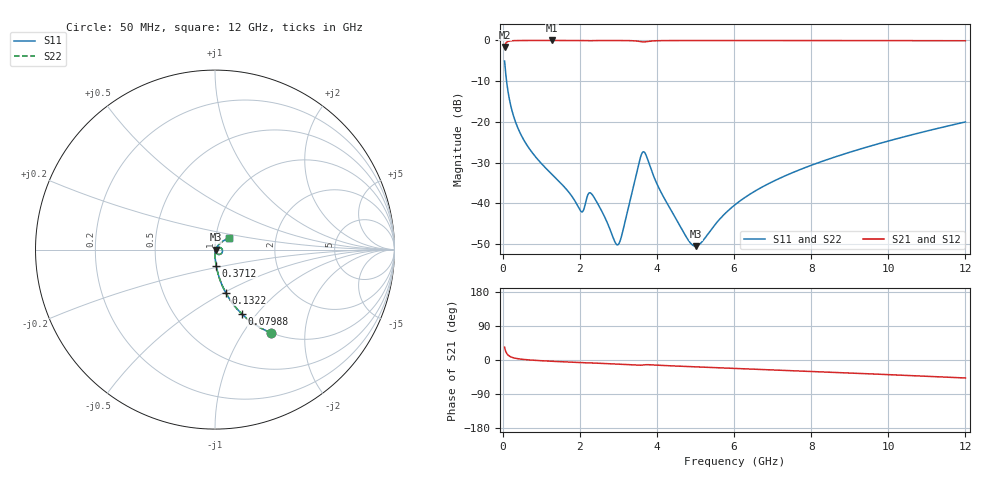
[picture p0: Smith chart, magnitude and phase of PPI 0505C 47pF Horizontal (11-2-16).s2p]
# MHz S MA R 50
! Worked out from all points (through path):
!   1601 points, 50 MHz to 12 GHz, reference 50 ohm
!   highest |S21| = -0.01 dB at 1.282 GHz (marker M1); lowest = -1.6 dB at 50 MHz (marker M2)
!   group delay of S21, straight-line fit = 11.7 ps
!   lowest |S11| = -50.5 dB at 5.002 GHz (marker M3), VSWR 1.01, Z = 50.3 - j0.0725 ohm
!   |S11| at or under -10 dB: 100.9 MHz to end of sweep
!   |S22| runs from -50.5 to -5.1 dB; largest |S21 - S12| = 0
!   S11 on the Smith chart (normalised r, x): 50 MHz: 1.00, -1.34; 79.88 MHz: 1.00, -0.84; 132.2 MHz: 1.00, -0.51; 371.2 MHz: 1.00, -0.18; 12 GHz: 1.15, +0.15
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50  0.5581 -56.2  0.8295 33.7  0.8295 33.7  0.5581 -56.2
79.875  0.3879 -67.4  0.9214 22.5  0.9214 22.5  0.3879 -67.4
132.1562  0.2463 -76.1  0.9688 13.8  0.9688 13.8  0.2463 -76.1
229.25  0.1446 -82.3  0.989 7.5  0.989 7.5  0.1446 -82.3
371.1562  0.08932 -85.8  0.9954 3.8  0.9954 3.8  0.08932 -85.8
714.7188  0.04517 -89.0  0.9981 -0.0  0.9981 -0.0  0.04517 -89.0
1282.344  0.02255 -90.7  0.9986 -3.4  0.9986 -3.4  0.02255 -90.7
2044.156  0.007861 -66.0  0.9958 -7.1  0.9958 -7.1  0.007861 -66.0
2223.406  0.01309 -52.8  0.9906 -7.6  0.9906 -7.6  0.01309 -52.8
2305.562  0.01305 -66.1  0.9929 -7.8  0.9929 -7.8  0.01305 -66.1
2977.75  0.003084 -19.1  0.9968 -10.8  0.9968 -10.8  0.003084 -19.1
3089.781  0.004069 17.7  0.9962 -11.3  0.9962 -11.3  0.004069 17.7
3620.062  0.04179 -6.1  0.9583 -13.4  0.9583 -13.4  0.04179 -6.1
3717.156  0.03909 -41.2  0.9653 -12.4  0.9653 -12.4  0.03909 -41.2
4038.312  0.01586 -76.0  0.9922 -13.8  0.9922 -13.8  0.01586 -76.0
4777.719  0.00375 -49.5  0.9965 -17.2  0.9965 -17.2  0.00375 -49.5
5001.781  0.002975 -14.0  0.9967 -18.1  0.9967 -18.1  0.002975 -14.0
6025  0.009589 51.2  0.9968 -22.2  0.9968 -22.2  0.009589 51.2
6854.031  0.01702 55.0  0.9966 -25.5  0.9966 -25.5  0.01702 55.0
8019.156  0.02948 54.0  0.9961 -30.3  0.9961 -30.3  0.02948 54.0
10013.31  0.05838 48.0  0.9943 -38.7  0.9943 -38.7  0.05838 48.0
12000  0.09973 40.2  0.9904 -47.5  0.9904 -47.5  0.09973 40.2
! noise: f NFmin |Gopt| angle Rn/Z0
50  0.0003817  0.8623  0.6075  0.0005943
1372  0.003918  0.6696  5.1  0.002275
2701  0.008737  0.7034  9.849  0.005736
4031  0.01742  0.7707  14.64  0.01524
5360  0.01243  0.6136  19.32  0.005816
6682  0.0138  0.5796  23.85  0.005732
8012  0.01559  0.5637  28.29  0.006078
9341  0.01751  0.5557  32.58  0.00655
1.067e+04  0.01953  0.5529  36.74  0.007098
1.2e+04  0.02166  0.5539  40.74  0.00772
